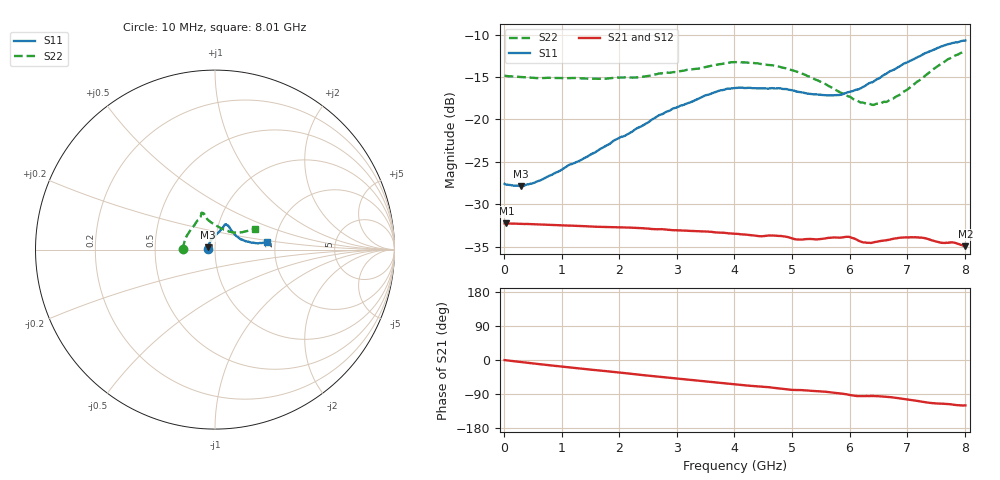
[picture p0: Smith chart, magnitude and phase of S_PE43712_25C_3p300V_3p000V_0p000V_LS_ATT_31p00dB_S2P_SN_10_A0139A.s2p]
! DEVICE ID: PE43712
! File Path: z:\PE43713\PE43713_CHAR_NOM_04292014\AMB\3p300\LS_ATT_31p00dB\PE43713_AMB_3p300V_3p000V_0p000V_LS_ATT_31p00dB_S2P_SN_10_A0139A.s2p
! Serial: 10
! Lot: A0139A
! Temp: 25C
! VDD: 3.300
! VSS: 0.000
! Control_Hi: 3.000
! Control_Lo: 0.000
! Attenuation Step: 31.00dB
! Port 1: RF1
! Port 2: RF2
! ThroughPath:1-2
! IDD: 0.0001457935
! ISS: 1.74e-008
#  Hz  S  RI  R  50
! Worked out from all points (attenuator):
!   801 points, 10 MHz to 8.01 GHz, reference 50 ohm
!   highest |S21| = -32.27 dB at 40 MHz (marker M1); lowest = -35.0 dB at 8.01 GHz (marker M2)
!   lowest |S11| = -27.9 dB at 290 MHz (marker M3), VSWR 1.08, Z = 46.3 + j1.23 ohm
!   |S11| at or under -10 dB: start of sweep to end of sweep
!   |S22| runs from -18.3 to -12.1 dB; largest |S21 - S12| = 0.00011
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1e7  -0.0417 0.0009  0.0243 -0.000108  0.0244 -0.000109  -0.1808 0.00126
4e7  -0.0411 0.00283  0.0243 -0.000336  0.0244 -0.000334  -0.18 0.00386
2.9e8  -0.0381 0.0133  0.0241 -0.00222  0.0241 -0.00222  -0.1767 0.0189
6.5e8  -0.0338 0.0281  0.0235 -0.00477  0.0235 -0.00478  -0.1704 0.0402
1.35e9  -0.021 0.054  0.0216 -0.00915  0.0216 -0.00913  -0.1556 0.0786
2.3e9  0.01 0.0877  0.0181 -0.0141  0.018 -0.0141  -0.1204 0.1292
2.68e9  0.0251 0.1024  0.0162 -0.0156  0.0162 -0.0156  -0.1037 0.1544
3.5e9  0.0484 0.1298  0.012 -0.0182  0.012 -0.0182  -0.079 0.1875
3.74e9  0.0533 0.138  0.0106 -0.0187  0.0106 -0.0187  -0.0763 0.1972
4.01e9  0.0582 0.1415  0.00916 -0.0191  0.00915 -0.0191  -0.0751 0.2042
4.76e9  0.0722 0.1345  0.00536 -0.0198  0.0054 -0.0199  -0.0599 0.1965
5.09e9  0.0821 0.1201  0.00366 -0.0192  0.00367 -0.0192  -0.0516 0.1836
5.35e9  0.0911 0.1073  0.0029 -0.0195  0.00285 -0.0194  -0.0439 0.1701
5.82e9  0.1143 0.0792  0.000629 -0.02  0.000671 -0.0201  -0.0116 0.1446
5.99e9  0.1269 0.0704  -0.0007 -0.0203  -0.00068 -0.0203  0.00387 0.1363
6.2e9  0.1414 0.0584  -0.00183 -0.0189  -0.00177 -0.0189  0.0261 0.123
6.41e9  0.1584 0.0514  -0.00161 -0.0187  -0.00159 -0.0187  0.05 0.1109
6.68e9  0.1852 0.0434  -0.00262 -0.0193  -0.00259 -0.0193  0.0826 0.0994
6.87e9  0.2017 0.039  -0.0039 -0.0197  -0.00387 -0.0196  0.1019 0.0952
7.22e9  0.233 0.0354  -0.00653 -0.019  -0.00651 -0.019  0.1412 0.0958
7.7e9  0.274 0.0391  -0.00822 -0.0168  -0.00819 -0.0168  0.1974 0.1088
8.01e9  0.2886 0.0432  -0.00887 -0.0155  -0.00882 -0.0156  0.2206 0.1161
